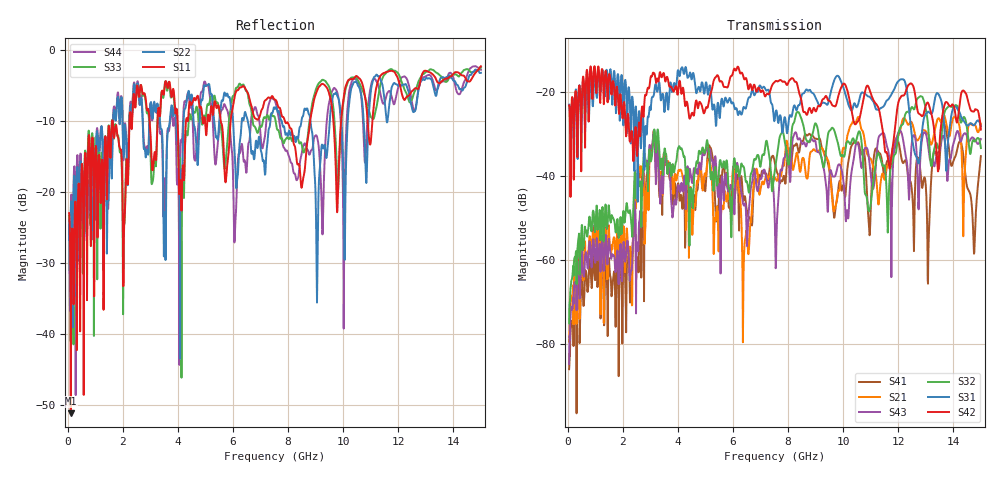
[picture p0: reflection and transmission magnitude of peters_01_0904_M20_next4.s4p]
# MHZ S RI R 50.00
! FREQ  S11  S12  S13  S14
!  S21  S22  S23  S24
!  S31  S32  S33  S34
!  S41  S42  S43  S44
!  REAL  IMAG  REAL  IMAG  REAL  IMAG  REAL  IMAG
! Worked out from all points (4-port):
!   1496 points, 50 MHz to 15 GHz, reference 50 ohm
!   strongest paths, dB at 50 MHz, 3.79 GHz, 7.53 GHz, 11.27 GHz, 15 GHz:
!     S42: -23.1, -19.1, -17.5, -23.6, -28.9
!     S31: -22.9, -19.8, -25.7, -24.2, -28.1
!     S32: -75.0, -38.4, -38.1, -34.5, -33.3
!     S43: -84.7, -49.0, -54.0, -31.3, -31.1
!     S21: -79.3, -39.3, -40.4, -46.4, -27.5
!     S41: -85.9, -41.4, -37.2, -34.2, -35.2
!   lowest |S11| = -51.2 dB at 110 MHz (marker M1), VSWR 1.01, Z = 50.2 - j0.152 ohm
!   |S11| at or under -10 dB: start of sweep to 1.616 GHz; 1.627 GHz to 2.243 GHz (616.5 MHz wide, 31.9 % of centre); 7.881 GHz to 8.802 GHz (920.8 MHz wide, 11 % of centre)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
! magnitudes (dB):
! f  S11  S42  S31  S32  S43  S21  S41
! 50 MHz  -23.0  -23.1  -22.9  -75.0  -84.7  -79.3  -85.9
! 110 MHz  -51.2  -34.4  -42.1  -66.2  -71.9  -70.1  -76.4
! 2.27 GHz  -8.8  -31.4  -25.7  -48.5  -63.8  -57.3  -69.9
! 3.1 GHz  -16.5  -15.3  -21.1  -31.9  -30.5  -31.2  -30.8
! 6.39 GHz  -5.1  -16.6  -23.5  -37.8  -46.9  -60.6  -45.6
! 7.94 GHz  -10.3  -18.2  -28.7  -33.9  -33.8  -31.6  -38.5
! 15 GHz  -2.3  -28.9  -28.1  -33.3  -31.1  -27.5  -35.2
